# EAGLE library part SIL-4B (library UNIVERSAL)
Rezistorova siet SIL 4xB
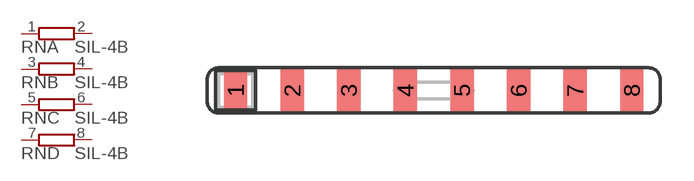
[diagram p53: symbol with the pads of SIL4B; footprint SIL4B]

Designator prefix RN; gates A=RNV B=RNV C=RNV D=RNV

## SIL-4B  [SIL4B]
1  A:1  pas
2  A:2  pas
3  B:1  pas
4  B:2  pas
5  C:1  pas
6  C:2  pas
7  D:1  pas
8  D:2  pas

## Footprint SIL4B (pad centres in mm)
smd 1.067 x 2.184: 1 -7.62,0; 2 -5.08,0; 3 -2.54,0; 4 0,0; 5 2.54,0; 6 5.08,0; 7 7.62,0; 8 10.16,0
